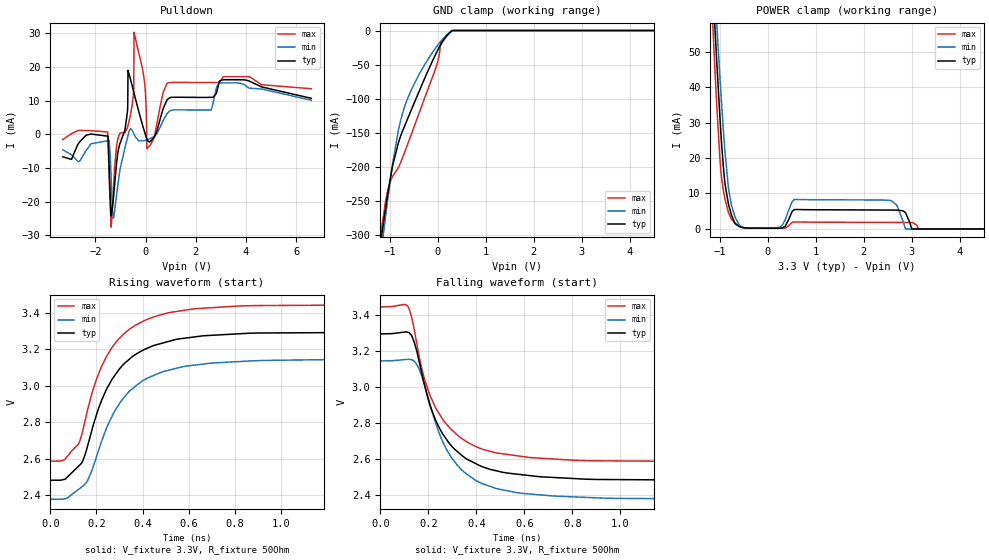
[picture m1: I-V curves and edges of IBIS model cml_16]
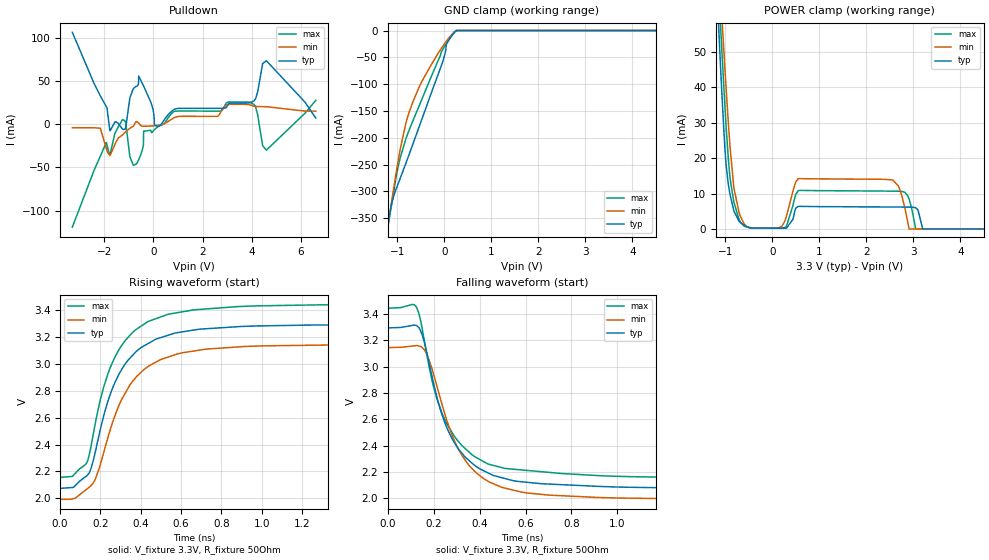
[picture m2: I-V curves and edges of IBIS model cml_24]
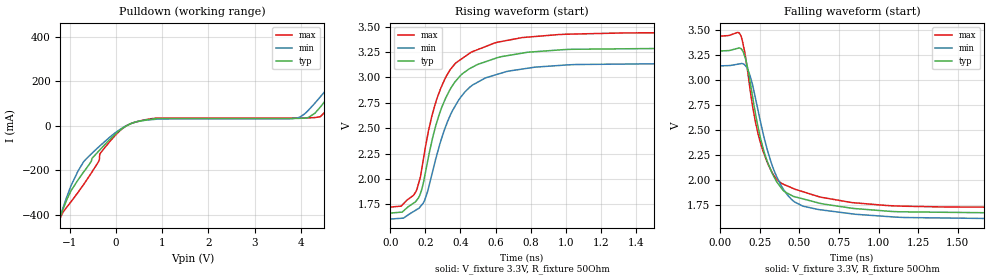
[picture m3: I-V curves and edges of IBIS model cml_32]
| Texas Instruments Incorporated
| LMK04832 Ultra Low-Noise JESD204B Compliant Clock Jitter Cleaner
| With Dual Loop PLLs
| Marketing part#   Digital Voltage Range   Package-type   #pins
| LMK04832   3.15 - 3.45V   WQFN   64
[IBIS Ver]   4.1
[File name]   lmk04832_industrial.ibs
[File Rev]   1.0
[Date]   18/12/2017
[Source]
| Texas Instruments Incorporated.
| Analog-eLab Design Center, HPA
| 12500 TI Blvd
| Dallas, TX -75243
[Notes]   Revision History:
| Rev 1.0: 18/12/2017
| - Initial version of the model
| - Model generated from simulations in SPECTRE
| - Model matched to SPICE simulation
| - C_comp although listed in numerical order of value are
|   obtained from varying PVT conditions. For PVT conditions for
|   each specific value refer the buffer description under
|   respective [Model]. IBIS model user is responsible for using
|   appropriate C_comp to simulate for Signal Integrity.
|* EXCEPTION:*
[Disclaimer]
| This model is designed as an aid for customers of Texas Instruments.
| TI and its licensors and suppliers make no warranties, either expressed
| or implied, with respect to this  model, including the warranties of
| merchantability or fitness for a particular purpose. The model is
| provided solely on an "as is" basis. The entire risk as to its quality
| and performance is with the customer.
[Copyright]
(C) Copyright 2017 Texas Instruments Incorporated.All rights reserved.
|   LMK04832
[Component]   LMK04832
[Manufacturer]   TI
[Package]   |64 WQFN
|   typ   min   max
R_pkg   0.067   0.027   0.083
L_pkg   0.937nH   0.593nH   1.143nH
C_pkg   0.144pF   0.126pF   0.200pF
[Pin]   signal_name   model_name   R_pin   L_pin   C_pin
1   CLKout0   clk_out_a2   NA   NA   NA
2   CLKout0*   clk_out_a2   NA   NA   NA
3   CLKout1   clk_out   NA   NA   NA
4   CLKout1*   clk_out   NA   NA   NA
5   RESET/GPO   io1   NA   NA   NA
6   SYNC/SYSREF_REQ   input1   NA   NA   NA
7   NC(VTHHI_EN)   input3   NA   NA   NA
8   NC(Fin)   nc   NA   NA   NA
9   NC(FinB)   nc   NA   NA   NA
10   Vcc1_VCO   power   NA   NA   NA
11   LDObyp1   nc   NA   NA   NA
12   LDObyp2   nc   NA   NA   NA
13   CLKout3   clk_out   NA   NA   NA
14   CLKout3*   clk_out   NA   NA   NA
15   CLKout2   clk_out_a2   NA   NA   NA
16   CLKout2*   clk_out_a2   NA   NA   NA
17   Vcc2_CG1   power   NA   NA   NA
18   CS*   input2   NA   NA   NA
19   SCK   input2   NA   NA   NA
20   SDIO   io2   NA   NA   NA
21   Vcc3_SYSREF   power   NA   NA   NA
22   CLKout5   clk_out   NA   NA   NA
23   CLKout5*   clk_out   NA   NA   NA
24   CLKout4   clk_out_a2   NA   NA   NA
25   CLKout4*   clk_out_a2   NA   NA   NA
26   Vcc4_CG2   power   NA   NA   NA
27   CLKout6   clk_out_a2   NA   NA   NA
28   CLKout6*   clk_out_a2   NA   NA   NA
29   CLKout7   clk_out   NA   NA   NA
30   CLKout7*   clk_out   NA   NA   NA
31   Status_LD1   io3   NA   NA   NA
32   CPout1   nc   NA   NA   NA
33   Vcc5_DIG   power   NA   NA   NA
34   CLKin1/FBCLKin/Fin1   nc   NA   NA   NA
35   CLKin1*/FBCLKin*/Fin18  nc   NA   NA   NA
36   Vcc6_PLL1   power   NA   NA   NA
37   CLKin0   nc   NA   NA   NA
38   CLKin0*   nc   NA   NA   NA
39   Vcc7_OSCout   power   NA   NA   NA
40   OSCout/CLKin2   osc_out   NA   NA   NA
41   OSCout*/CLKin2*   osc_out   NA   NA   NA
42   Vcc8_OSCin   power   NA   NA   NA
43   OSCin   nc   NA   NA   NA
44   OSCin*   nc   NA   NA   NA
45   Vcc9_CP2   power   NA   NA   NA
46   CPout2   nc   NA   NA   NA
47   Vcc10_PLL2   power   NA   NA   NA
48   Status_LD2   io4   NA   NA   NA
49   CLKout9   clk_out   NA   NA   NA
50   CLKout9*   clk_out   NA   NA   NA
51   CLKout8   clk_out   NA   NA   NA
52   CLKout8*   clk_out   NA   NA   NA
53   Vcc11_CG3   power   NA   NA   NA
54   CLKout10   clk_out   NA   NA   NA
55   CLKout10*   clk_out   NA   NA   NA
56   CLKout11   clk_out   NA   NA   NA
57   CLKout11*   clk_out   NA   NA   NA
58   CLKin_SEL0   io1   NA   NA   NA
59   CLKin_SEL1   io1   NA   NA   NA
60   CLKout13   clk_out   NA   NA   NA
61   CLKout13*   clk_out   NA   NA   NA
62   CLKout12   clk_out_a2   NA   NA   NA
63   CLKout12*   clk_out_a2   NA   NA   NA
64   Vcc12_CG0   power   NA   NA   NA
|   Model Selectors
[Model Selector] clk_out
cml_16   3.3V   Open_drain
cml_24   3.3V   Open_drain
cml_32   3.3V   Open_drain
hsds_6   3.3V   3-state
hsds_8   3.3V   3-state
lcpecl   3.3V   Output
lvcmos   3.3V   3-state
LVDS_CO   3.3V   Output
LVPECL16_CO   3.3V   Output
LVPECL20_CO   3.3V   Output
|lcpecl   3.3V   Output
[Model Selector] clk_out_a2
cml_16   3.3V   Open_drain
cml_24   3.3V   Open_drain
cml_32   3.3V   Open_drain
hsds_6   3.3V   3-state
hsds_8   3.3V   3-state
lcpecl   3.3V   Output
LVDS_CO   3.3V   Output
LVPECL16_CO   3.3V   Output
LVPECL20_CO   3.3V   Output
[Model Selector] osc_out
diffio_lvcmos   3.3V   I/O
diffio_lvds   3.3V   I/O
diffio_lvpecl_16   3.3V   I/O
diffio_lvpecl_20   3.3V   I/O
| Models and submodels in the file (21): cml_16 (Open_drain), cml_24 (Open_drain), cml_32 (Open_drain), diffio_lvcmos (I/O), diffio_lvds (I/O), diffio_lvpecl_16 (I/O), diffio_lvpecl_20 (I/O), hsds_6 (3-state), hsds_8 (3-state), input1 (Input), input2 (Input), input3 (Input), io1 (I/O), io2 (I/O), io3 (I/O), io4 (I/O), lcpecl (Output), lvcmos (Output), LVDS_CO (Output), LVPECL16_CO (Output), LVPECL20_CO (Output)
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|   cml_16 Model
[Model]   cml_16
Model_type   Open_drain
Polarity   Non-Inverting
Vmeas = 2.8
Vref = 3.3
Cref = 1pF
Rref = 50
|   typ   min   max
C_comp   2.136pF   2.117pF   2.176pF
|  Where Nom  PVT is Nominal Process,   3.3V,  25C
|   Fast PVT is Strong Process,   3.45V, -40C
|   Slow PVT is Weak Process,   3.15V, 85C
[Voltage Range]   3.3   3.15   3.45
|Junction Temperature
[Temperature Range]   25   85   -40
[Pullup Reference]   3.3   3.15   3.45
[Pulldown Reference]   0   0   0
[Power Clamp Reference]   3.3   3.15   3.45
[GND Clamp Reference]   0   0   0
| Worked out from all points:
|   slope of the pulldown table from 0 to 0.495 V, typ, clamps not added: 205 ohm
|   POWER clamp passes 1 mA (typ) near -0.63 V on its own axis
|   falling waveform, V_fixture 3.3V, R_fixture 50Ohm: 20-80 % time 155ps typ, 158ps min, 154ps max; typ from 3.29 V to 2.48 V
|   rising waveform, V_fixture 3.3V, R_fixture 50Ohm: 20-80 % time 174ps typ, 185ps min, 169ps max; typ from 2.48 V to 3.29 V
[Pulldown]
|   Voltage   I(typ)   I(min)   I(max)
-3.3V     -6.645mA   -4.572mA   -1.54mA
-1.51V    -524.3uA   -1.877mA   712.1uA
-1.37V    -24.21mA   -13.11mA   -27.56mA
-1.15V    -8.102mA   -17.72mA   -3.121mA
-720mV    6.846mA    -1.057mA   2.077mA
-700mV    19.08mA    -413.4uA   2.635mA
-490mV    13.13mA    607.8uA    11.42mA
-460mV    12.24mA    112.2uA    30.33mA
-40mV     736.1uA    -1.83mA    15.49mA
50mV      -1.435mA   -1.628mA   -4.2mA
860mV     10.36mA    6.207mA    15.25mA
6.6V      10.72mA    10.15mA    13.57mA
[GND Clamp]
|   Voltage   I(typ)   I(min)   I(max)
-3.3V     -1.623A    -1.546A    -1.728A
-1.25V    -343.9mA   -365.3mA   -333.5mA
-1.16V    -295.3mA   -312.9mA   -284.3mA
-1.1V     -265.9mA   -278.7mA   -255.3mA
-1V       -220.9mA   -224mA     -223.7mA
-820mV    -164.3mA   -145.4mA   -201.1mA
-680mV    -137.9mA   -109.2mA   -176.3mA
-400mV    -90.84mA   -65.49mA   -123mA
-50mV     -35.52mA   -26.05mA   -56.37mA
50mV      -21.71mA   -16.84mA   -22.44mA
290mV     -707.9uA   0A         -978.3uA
6.6V      0A         0A         0A
[POWER Clamp]
|   Voltage   I(typ)   I(min)   I(max)
-3.3V     686.9mA    636.8mA    746.8mA
-1.17V    74.27mA    82.81mA    64.08mA
-1.1V     55.92mA    65.93mA    44.03mA
-1.07V    48.34mA    58.89mA    35.98mA
-980mV    27.38mA    38.7mA     16.58mA
-890mV    12.44mA    21.14mA    8.242mA
-760mV    3.997mA    6.769mA    2.767mA
-590mV    633.6uA    1.041mA    826.7uA
550mV     5.41mA     8.314mA    1.961mA
2.4V      5.334mA    8.151mA    1.851mA
2.87V     4.589mA    0A         1.833mA
6.6V      0A         0A         0A
[Ramp]
R_load = 50
|   typ   min   max
dV/dt_r   0.487874/1.73824e-10   0.4608/1.8331e-10   0.514985/1.67857e-10
dV/dt_f   0.487821/1.54217e-10   0.460763/1.57982e-10   0.514909/1.52704e-10
[Falling Waveform]
V_fixture = 3.3V
V_fixture_min = 3.15V
V_fixture_max = 3.45V
R_fixture = 50Ohm
C_fixture = 0F
|   Time   V(typ)   V(min)   V(max)
0s        3.295V     3.146V     3.445V
115.1ps   3.304V     3.155V     3.448V
132.5ps   3.281V     3.151V     3.376V
159.9ps   3.154V     3.107V     3.185V
207.7ps   2.898V     2.902V     2.953V
256.4ps   2.749V     2.708V     2.828V
328ps     2.635V     2.556V     2.726V
484.8ps   2.535V     2.437V     2.635V
811.3ps   2.493V     2.391V     2.594V
20ns      2.482V     2.378V     2.587V
[Rising Waveform]
V_fixture = 3.3V
V_fixture_min = 3.15V
V_fixture_max = 3.45V
R_fixture = 50Ohm
C_fixture = 0F
|   Time   V(typ)   V(min)   V(max)
0s        2.482V     2.378V     2.587V
61.19ps   2.487V     2.38V      2.594V
121.5ps   2.558V     2.431V     2.679V
156.9ps   2.648V     2.472V     2.842V
220.8ps   2.915V     2.691V     3.102V
274.3ps   3.048V     2.85V      3.222V
328ps     3.13V      2.949V     3.295V
484.8ps   3.233V     3.076V     3.39V
811.3ps   3.284V     3.132V     3.436V
20ns      3.295V     3.146V     3.445V
|   cml_24 Model
[Model]   cml_24
Model_type   Open_drain
Polarity   Non-Inverting
Vmeas = 2.7
Vref = 3.3
Cref = 1pF
Rref = 50
|   typ   min   max
C_comp   2.136pF   2.117pF   2.176pF
|  Where Nom  PVT is Nominal Process,   3.3V,  25C
|   Fast PVT is Strong Process,   3.45V, -40C
|   Slow PVT is Weak Process,   3.15V, 85C
[Voltage Range]   3.3   3.15   3.45
|Junction Temperature
[Temperature Range]   25   85   -40
[Pullup Reference]   3.3   3.15   3.45
[Pulldown Reference]   0   0   0
[Power Clamp Reference]   3.3   3.15   3.45
[GND Clamp Reference]   0   0   0
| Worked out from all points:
|   POWER clamp passes 1 mA (typ) near -0.60 V on its own axis
|   falling waveform, V_fixture 3.3V, R_fixture 50Ohm: 20-80 % time 158ps typ, 165ps min, 157ps max; typ from 3.29 V to 2.07 V
|   rising waveform, V_fixture 3.3V, R_fixture 50Ohm: 20-80 % time 180ps typ, 190ps min, 173ps max; typ from 2.07 V to 3.29 V
[Pulldown]
|   Voltage   I(typ)   I(min)   I(max)
-3.3V     106.4mA    -4.09mA    -119.2mA
-2.16V    32.73mA    -4.641mA   -36.98mA
-1.77V    -7.458mA   -35.9mA    -35.96mA
-1.25V    -5.986mA   -12.21mA   5.363mA
-820mV    41.24mA    -2.338mA   -47.54mA
-600mV    55.74mA    1.138mA    -40.94mA
-400mV    44.18mA    -2.337mA   -8.101mA
160mV     -2.368mA   -1.367mA   -3.293mA
3.1V      24.33mA    23mA       25.77mA
4.13V     28.48mA    20.66mA    21.09mA
4.59V     73.42mA    20.25mA    -29.95mA
6.6V      7.131mA    15.09mA    27.54mA
[GND Clamp]
|   Voltage   I(typ)   I(min)   I(max)
-3.3V     -1.726A    -1.54A     -1.613A
-1.24V    -379.2mA   -382.9mA   -384.9mA
-1.12V    -321.3mA   -316.7mA   -321.4mA
-980mV    -284.6mA   -240.1mA   -251.7mA
-820mV    -247.4mA   -172.5mA   -201.7mA
-760mV    -233mA     -154.8mA   -187.5mA
-490mV    -167.6mA   -96.6mA    -130.1mA
-50mV     -61.33mA   -31.18mA   -37.5mA
20mV      -40.08mA   -22.41mA   -26.96mA
40mV      -26.15mA   -20.04mA   -24.13mA
240mV     -788uA     -151.8uA   -1.027mA
6.6V      0A         0A         0A
[POWER Clamp]
|   Voltage   I(typ)   I(min)   I(max)
-3.3V     749.5mA    639mA      689.4mA
-1.2V     73.76mA    89.78mA    82.99mA
-1.08V    39.57mA    61.21mA    51.67mA
-900mV    9.721mA    23.11mA    14.36mA
-600mV    1.026mA    1.407mA    794.8uA
200mV     214.1uA    771.6uA    259.1uA
550mV     6.359mA    14.24mA    10.8mA
2.26V     6.226mA    14.05mA    10.72mA
2.68V     6.197mA    12.19mA    10.67mA
2.91V     6.18mA     0A         8.494mA
3.05V     6.013mA    0A         0A
6.6V      0A         0A         0A
[Ramp]
R_load = 50
|   typ   min   max
dV/dt_r   0.732563/1.78381e-10   0.691882/1.90134e-10   0.773274/1.72328e-10
dV/dt_f   0.732469/1.57582e-10   0.691812/1.64005e-10   0.773149/1.56138e-10
[Falling Waveform]
V_fixture = 3.3V
V_fixture_min = 3.15V
V_fixture_max = 3.45V
R_fixture = 50Ohm
C_fixture = 0F
|   Time   V(typ)   V(min)   V(max)
0s        3.294V     3.145V     3.444V
122.8ps   3.312V     3.16V      3.455V
165ps     3.136V     3.108V     3.132V
196.3ps   2.89V      2.956V     2.861V
231.2ps   2.657V     2.739V     2.665V
296.6ps   2.402V     2.409V     2.454V
366.9ps   2.266V     2.224V     2.33V
584ps     2.125V     2.046V     2.215V
933.4ps   2.089V     2.005V     2.171V
20ns      2.073V     1.992V     2.155V
[Rising Waveform]
V_fixture = 3.3V
V_fixture_min = 3.15V
V_fixture_max = 3.45V
R_fixture = 50Ohm
C_fixture = 0F
|   Time   V(typ)   V(min)   V(max)
0s        2.073V     1.992V     2.155V
60.35ps   2.08V      1.995V     2.162V
132.3ps   2.167V     2.068V     2.265V
174.9ps   2.349V     2.143V     2.562V
236.6ps   2.721V     2.45V      2.926V
296.6ps   2.937V     2.709V     3.119V
359.1ps   3.065V     2.87V      3.235V
584ps     3.235V     3.076V     3.384V
881ps     3.278V     3.127V     3.428V
20ns      3.294V     3.145V     3.444V
|   cml_32 Model
[Model]   cml_32
Model_type   Open_drain
Polarity   Non-Inverting
Vmeas = 2.5
Vref = 3.3
Cref = 1pF
Rref = 50
|   typ   min   max
C_comp   2.136pF   2.117pF   2.176pF
|  Where Nom  PVT is Nominal Process,   3.3V,  25C
|   Fast PVT is Strong Process,   3.45V, -40C
|   Slow PVT is Weak Process,   3.15V, 85C
[Voltage Range]   3.3   3.15   3.45
|Junction Temperature
[Temperature Range]   25   85   -40
[Pullup Reference]   3.3   3.15   3.45
[Pulldown Reference]   0   0   0
[Power Clamp Reference]   3.3   3.15   3.45
[GND Clamp Reference]   0   0   0
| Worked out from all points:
|   slope of the pulldown table from 0 to 0.495 V, typ, clamps not added: 8.9 ohm
|   falling waveform, V_fixture 3.3V, R_fixture 50Ohm: 20-80 % time 162ps typ, 175ps min, 157ps max; typ from 3.29 V to 1.67 V
|   rising waveform, V_fixture 3.3V, R_fixture 50Ohm: 20-80 % time 182ps typ, 197ps min, 176ps max; typ from 1.67 V to 3.29 V
[Pulldown]
|   Voltage   I(typ)   I(min)   I(max)
-3.3V     -1.611A    -1.541A    -1.728A
-1.26V    -441.4mA   -433.7mA   -440.8mA
-970mV    -291mA     -268mA     -340.7mA
-700mV    -207.6mA   -161.9mA   -264mA
-260mV    -88.74mA   -73.99mA   -103mA
370mV     13.25mA    13.34mA    13.3mA
880mV     31.83mA    29.45mA    34.3mA
3.81V     32.9mA     31.87mA    34.73mA
4.16V     37.2mA     69.56mA    35.37mA
4.42V     84.4mA     130.2mA    40.97mA
5.24V     310.8mA    337.7mA    277.1mA
6.6V      702.6mA    693.5mA    713.7mA
[Ramp]
R_load = 50
|   typ   min   max
dV/dt_r   0.977234/1.81256e-10   0.922927/1.96831e-10   1.03156/1.74054e-10
dV/dt_f   0.977116/1.61742e-10   0.922841/1.74865e-10   1.0314/1.56594e-10
[Falling Waveform]
V_fixture = 3.3V
V_fixture_min = 3.15V
V_fixture_max = 3.45V
R_fixture = 50Ohm
C_fixture = 0F
|   Time   V(typ)   V(min)   V(max)
0s        3.293V     3.144V     3.443V
130.9ps   3.318V     3.166V     3.449V
161.6ps   3.209V     3.142V     3.221V
187.5ps   3.002V     3.054V     2.928V
242.3ps   2.51V      2.676V     2.445V
297.1ps   2.187V     2.305V     2.179V
358.2ps   1.977V     2.028V     2.002V
522.3ps   1.808V     1.735V     1.88V
1.053ns   1.685V     1.631V     1.741V
20ns      1.665V     1.606V     1.724V
[Rising Waveform]
V_fixture = 3.3V
V_fixture_min = 3.15V
V_fixture_max = 3.45V
R_fixture = 50Ohm
C_fixture = 0F
|   Time   V(typ)   V(min)   V(max)
0s        1.665V     1.606V     1.723V
63.13ps   1.673V     1.613V     1.734V
161.6ps   1.816V     1.71V      1.958V
196.9ps   2.034V     1.795V     2.28V
256.1ps   2.504V     2.177V     2.738V
306.6ps   2.761V     2.475V     2.967V
369.3ps   2.958V     2.717V     3.135V
542.2ps   3.154V     2.995V     3.304V
956.7ps   3.27V      3.117V     3.422V
20ns      3.293V     3.144V     3.443V
